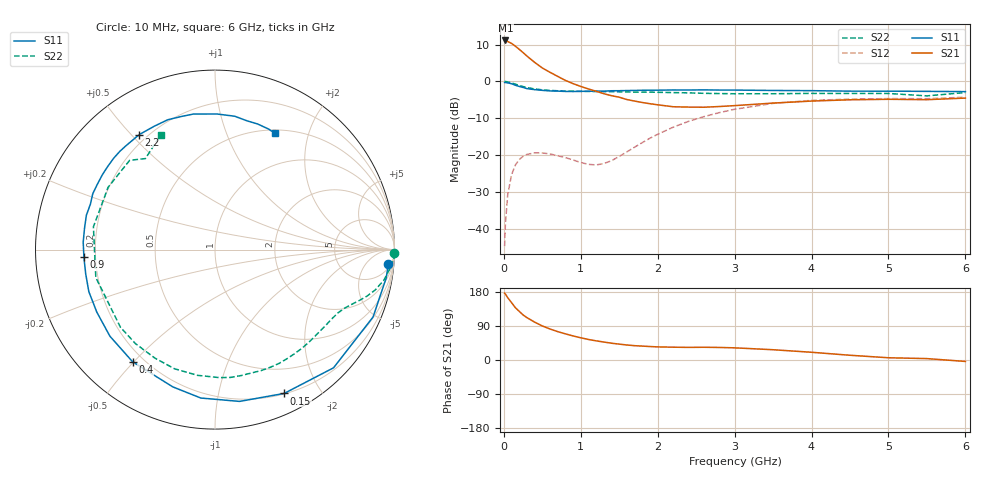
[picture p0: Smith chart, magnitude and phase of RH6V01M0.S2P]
! SIEMENS Small Signal Semiconductors
! BFR106
! Si NPN RF Bipolar Junction Transistor in SOT23
! VCE = 6 V  IC = 1 mA
! Common Emitter S-Parameters:  August  1996
# GHz  S  MA  R  50
!  f  S11  S21  S12  S22
! GHz  MAG  ANG  MAG  ANG  MAG  ANG  MAG  ANG
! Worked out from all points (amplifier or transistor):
!   36 points, 10 MHz to 6 GHz, reference 50 ohm
!   highest |S21| = 11.1 dB at 20 MHz (marker M1)
!   |S21| within 3 dB of that: start of sweep to 234 MHz
!   unconditionally stable (mu >= 1): 861.6 MHz to 1.891 GHz; 3.051 GHz to end of sweep
!   at 250 MHz: K = 0.26, MSG = 14.0 dB, |S12| = -20.3 dB
!   at 1.4 GHz: K = 1.39, MAG = 5.1 dB, |S12| = -21.4 dB
!   at 6 GHz: K = 1.02, MAG = -0.9 dB, |S12| = -4.3 dB
!   S11 on the Smith chart (normalised r, x): 10 MHz: 8, -21; 150 MHz: 0.21, -1.57; 400 MHz: 0.16, -0.50; 900 MHz: 0.16, -0.03; 2.2 GHz: 0.17, +0.53; 6 GHz: 0.54, +1.50
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0.01  0.9692 -4.8  3.589 176.3  0.0059 89.8  0.9999 -1.2
0.02  0.9669 -9.4  3.59 174.1  0.0117 84.0  1 -2.3
0.05  0.9573 -23.1  3.478 164.5  0.0291 77.0  0.9859 -5.4
0.1  0.9328 -44.9  3.28 151.5  0.0546 65.4  0.9568 -10.2
0.15  0.8892 -64.3  3 138.1  0.074 54.7  0.92 -14.2
0.2  0.8568 -80.8  2.723 128.4  0.0877 46.8  0.8857 -17.0
0.25  0.8307 -95.5  2.46 118.9  0.097 39.5  0.8528 -19.4
0.3  0.8002 -107.1  2.208 111.8  0.103 34.7  0.8284 -21.2
0.4  0.7755 -126.3  1.815 100.0  0.1079 26.6  0.7924 -24.3
0.5  0.7587 -140.5  1.523 89.9  0.1077 21.6  0.7702 -27.3
0.6  0.745 -152.1  1.331 81.8  0.1046 18.8  0.7572 -30.5
0.9  0.7315 -176.6  0.935 63.5  0.0866 20.9  0.7373 -40.7
1.1  0.7368 170.5  0.792 54.2  0.0755 32.9  0.733 -48.5
1.3  0.739 159.9  0.683 47.4  0.0774 52.2  0.7283 -56.4
1.6  0.7536 146.3  0.569 39.6  0.1116 74.0  0.7213 -69.2
2.2  0.7673 123.4  0.455 33.8  0.2402 76.4  0.7073 -97.9
2.8  0.765 104.2  0.458 33.1  0.3784 62.2  0.6861 -130.2
3.5  0.7556 89.1  0.51 27.1  0.5053 43.2  0.682 -166.8
4.5  0.7393 76.0  0.565 12.5  0.5768 19.4  0.6894 149.8
5  0.7391 71.2  0.574 5.9  0.5866 10.6  0.688 133.7
5.5  0.7348 65.9  0.567 3.7  0.5849 6.4  0.6383 127.4
6  0.7287 62.8  0.596 -3.8  0.6126 -1.8  0.7076 115.3
